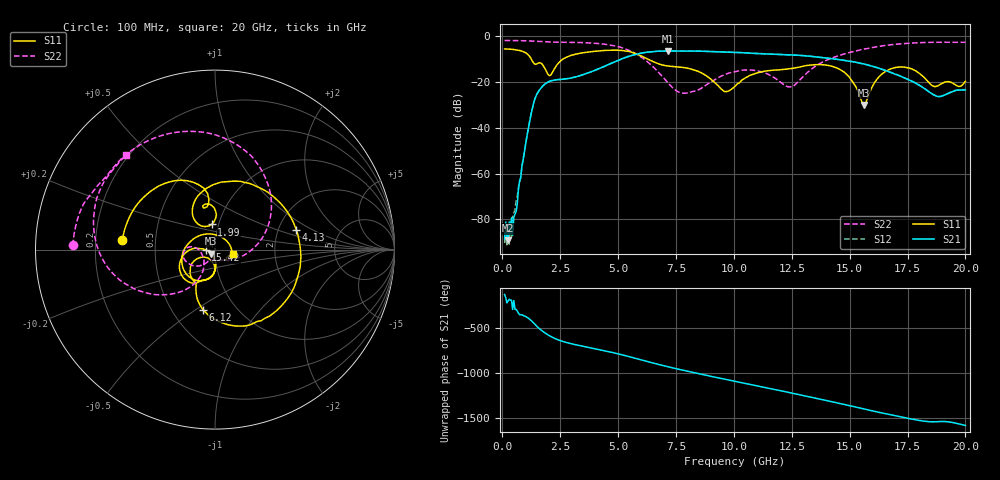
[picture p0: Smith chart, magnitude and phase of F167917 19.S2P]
!  2-Port S-parameters saved by WinCal
! VAR MeasName=S-Parameters (CALIBRATED_DATA) read from VNA (N5242A)
! VAR MeasDate=2016-11-22 9:00:39
! VAR NAME=F167917 19
! VAR FILENAME=F167917 19.S2P
! VAR DATE=2016-11-22 9:00:39
! VAR PHYS_PORTS=1,2
# Hz S DB R 50
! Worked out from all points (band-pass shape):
!   401 points, 100 MHz to 20 GHz, reference 50 ohm
!   highest |S21| = -6.61 dB at 7.165 GHz (marker M1); lowest = -89.2 dB at 249.2 MHz (marker M2)
!   |S21| within 3 dB of the highest: 5.266 GHz to 13.91 GHz (8.643 GHz wide, 90.2 % of centre)
!   lowest |S11| = -30.1 dB at 15.62 GHz (marker M3), VSWR 1.06, Z = 47.8 - j2.13 ohm
!   |S11| at or under -10 dB: 1.245 GHz to 2.642 GHz (1.397 GHz wide, 71.9 % of centre); 6.253 GHz to end of sweep
!   |S22| runs from -25.0 to -2.0 dB; largest |S21 - S12| = 0.0044
!   S11 on the Smith chart (normalised r, x): 100 MHz: 0.32, +0.05; 1.99 GHz: 0.93, +0.27; 4.13 GHz: 2.52, +0.70; 6.12 GHz: 0.71, -0.54; 15.42 GHz: 0.90, -0.00; 20 GHz: 1.22, -0.06
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1e8  -5.71 174.2  -88.52 -130.7  -90.29 155.9  -2.03 178.3
2.4925e8  -5.78 165.4  -89.15 156.4  -82.00 160.4  -2.04 175.8
5.4775e8  -6.05 147.4  -77.74 65.9  -76.06 79.2  -2.07 170.9
1.3935e9  -12.31 100.6  -27.94 -97.2  -27.91 -97.3  -2.39 156.7
1.9905e9  -17.00 97.6  -20.07 138.4  -20.05 138.3  -2.68 147.9
3.43325e9  -7.50 56.6  -17.13 16.6  -17.13 16.4  -2.95 121.7
4.12975e9  -6.63 13.5  -14.50 -20.0  -14.52 -20.1  -3.37 103.9
5.274e9  -6.52 -57.0  -9.58 -87.4  -9.56 -87.2  -5.56 62.3
6.11975e9  -9.34 -101.1  -7.35 -145.5  -7.32 -145.6  -10.13 21.8
6.7665e9  -12.26 -115.9  -6.70 170.9  -6.69 170.9  -16.12 -13.4
7.1645e9  -13.18 -119.0  -6.61 145.7  -6.60 145.7  -20.58 -38.7
8.40825e9  -15.28 -143.2  -6.69 73.4  -6.66 73.4  -23.74 -117.2
1.005e10  -22.01 -95.6  -7.22 -16.1  -7.22 -16.0  -15.61 -152.2
1.1244e10  -15.58 -102.3  -7.82 -79.2  -7.79 -79.0  -15.82 177.9
1.2438e10  -14.31 -115.2  -8.35 -142.4  -8.31 -142.5  -22.26 -153.5
1.338325e10  -12.68 -129.6  -9.01 164.8  -8.97 164.9  -14.25 -119.4
1.467675e10  -15.23 -171.6  -10.57 92.4  -10.55 92.3  -8.18 -139.8
1.5423e10  -25.79 -178.2  -11.88 49.0  -11.88 49.0  -6.21 -152.5
1.5622e10  -30.14 -134.4  -12.28 37.2  -12.33 37.4  -5.80 -156.0
1.67165e10  -14.64 -111.3  -15.70 -25.7  -15.67 -25.2  -3.98 -175.9
1.875625e10  -21.99 44.4  -26.32 -105.4  -26.23 -104.8  -2.80 149.7
2e10  -19.83 -14.7  -23.59 -146.4  -23.48 -146.1  -2.82 133.5
